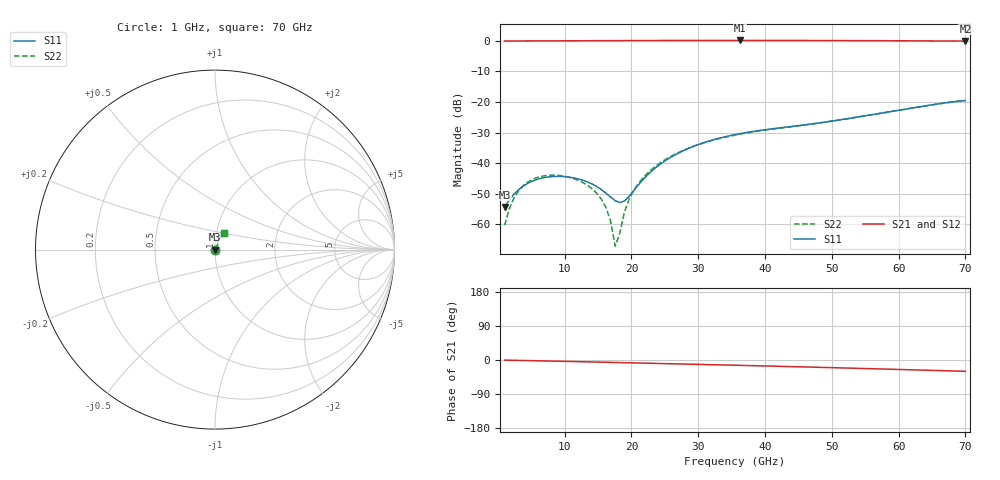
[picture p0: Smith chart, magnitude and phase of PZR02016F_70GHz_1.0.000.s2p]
# GHz S RI R 50
! S-Parameters data
! Freq  reS11  imS11  reS21  imS21  reS12  imS12  reS22  imS22
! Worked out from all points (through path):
!   101 points, 1 GHz to 70 GHz, reference 50 ohm
!   highest |S21| = 0.15 dB at 36.19 GHz (marker M1); lowest = -0.1 dB at 70 GHz (marker M2)
!   group delay of S21, straight-line fit = 1.19 ps
!   lowest |S11| = -54.4 dB at 1 GHz (marker M3), VSWR 1.00, Z = 50.2 - j0.0656 ohm
!   |S11| at or under -10 dB: start of sweep to end of sweep
!   |S22| runs from -67.2 to -19.5 dB; largest |S21 - S12| = 0
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1  0.00179 -0.000653  0.9993 -0.00648  0.9993 -0.00648  -0.000453 -0.000848
1.69  0.00193 -0.00157  0.9991 -0.0107  0.9991 -0.0107  -0.00035 -0.00172
2.38  0.00179 -0.0025  0.9992 -0.0147  0.9992 -0.0147  -0.000448 -0.00262
3.76  0.00106 -0.00403  0.9996 -0.0229  0.9996 -0.0229  -0.00101 -0.00411
5.14  6.06e-05 -0.00505  1 -0.0315  1 -0.0315  -0.00173 -0.00509
8.59  -0.00215 -0.00565  1.002 -0.0536  1.002 -0.0536  -0.0029 -0.00562
12.73  -0.00328 -0.00406  1.003 -0.0813  1.003 -0.0813  -0.00254 -0.00405
14.8  -0.00321 -0.00259  1.004 -0.0955  1.004 -0.0955  -0.00183 -0.00263
16.18  -0.00291 -0.00137  1.004 -0.1052  1.004 -0.1052  -0.00119 -0.00144
16.87  -0.00269 -0.000681  1.004 -0.11  1.004 -0.11  -0.000824 -0.000767
17.56  -0.00242 5.29e-05  1.004 -0.1149  1.004 -0.1149  -0.000433 -5.07e-05
18.25  -0.0021 0.000833  1.004 -0.1198  1.004 -0.1198  -1.36e-05 0.000712
18.94  -0.00172 0.00166  1.004 -0.1247  1.004 -0.1247  0.000431 0.00152
20.32  -0.000822 0.00343  1.004 -0.1346  1.004 -0.1346  0.00139 0.00326
22.39  0.000883 0.00632  1.003 -0.1495  1.003 -0.1495  0.00299 0.00613
24.46  0.00294 0.00942  1.002 -0.1644  1.002 -0.1644  0.00469 0.00922
29.29  0.00831 0.0168  0.997 -0.1991  0.997 -0.1991  0.00857 0.0168
35.5  0.0141 0.0256  0.9877 -0.2434  0.9877 -0.2434  0.0123 0.0259
36.19  0.0146 0.0264  0.9865 -0.2484  0.9865 -0.2484  0.0126 0.0268
47.23  0.0177 0.0404  0.9598 -0.3294  0.9598 -0.3294  0.0162 0.0408
58.96  0.0269 0.0646  0.9161 -0.4164  0.9161 -0.4164  0.0283 0.064
70  0.0496 0.0933  0.8615 -0.4958  0.8615 -0.4958  0.0491 0.0934
